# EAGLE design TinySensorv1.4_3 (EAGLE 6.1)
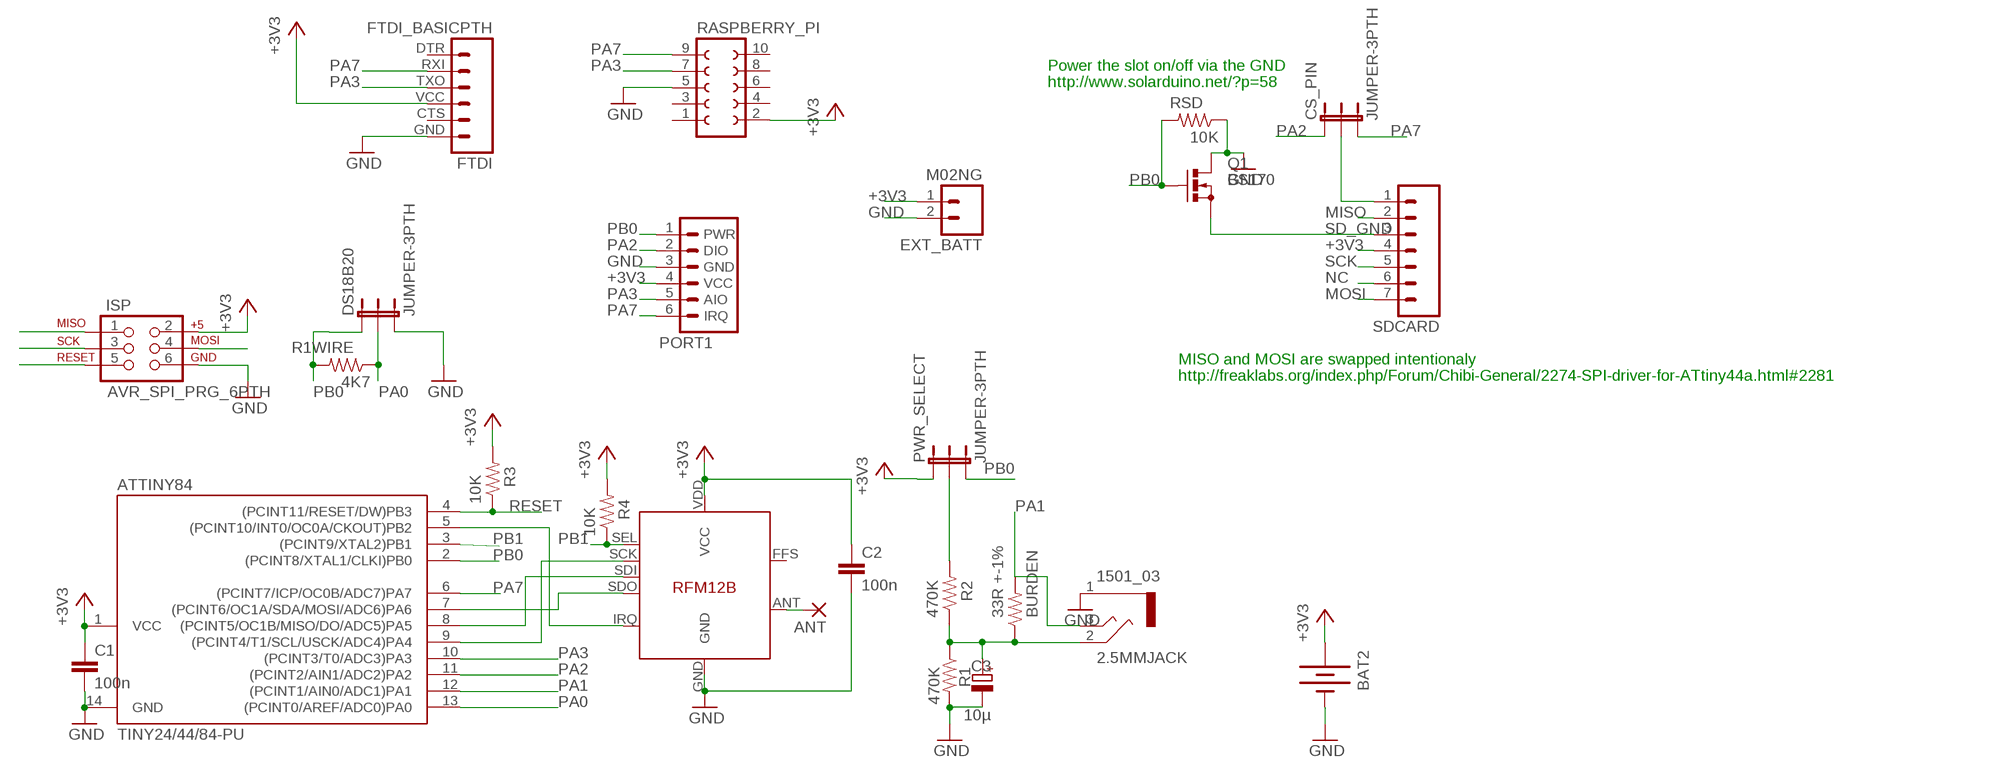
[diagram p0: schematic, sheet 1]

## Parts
2.5MMJACK  1501_03  [1501_03]
ANT  1,6/0,8  [1,6/0,8]
ATTINY84  TINY24/44/84-PU  [DIL14]
BAT2  BATTERY20PTH  [BATTCOM_20MM_PTH]
BURDEN  33R +-1%  RESISTORAXIAL-0.3  [AXIAL-0.3]
C1  100n  C-EU025-024X044  [C025-024X044]
C2  100n  C-EU025-024X044  [C025-024X044]
C3  10µ  CPOL-EUE2.5-6  [E2,5-6]
CS_PIN  JUMPER-3PTH  [1X03]
DS18B20  JUMPER-3PTH  [1X03]
EXT_BATT  M02NG  [1X02]
FTDI  FTDI_BASICPTH  [FTDI_BASIC]
ISP  AVR_SPI_PRG_6PTH  [2X3]
PORT1  JEEPORT-FEMALE  [1X06_FEMALE_LOCK.010]
PWR_SELECT  JUMPER-3PTH  [1X03]
Q1  BS170  [SOT54E]
R1  470K  RESISTORAXIAL-0.3  [AXIAL-0.3]
R1WIRE  4K7  RESISTORAXIAL-0.3  [AXIAL-0.3]
R2  470K  RESISTORAXIAL-0.3  [AXIAL-0.3]
R3  10K  RESISTORAXIAL-0.3  [AXIAL-0.3]
R4  10K  RESISTORAXIAL-0.3  [AXIAL-0.3]
RASPBERRY_PI  FE05-2  [FE05-2]
RFM12B  RFM12B  [RFM12B]
RSD  10K  RESISTORAXIAL-0.3  [AXIAL-0.3]
SDCARD  M07LOCK  [1X07_LOCK]

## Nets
+3V3 [power]: ATTINY84.1(VCC) BAT2.1(+) C1.1 C2.1 EXT_BATT.1 FTDI.VCC ISP.2 PORT1.4(VCC) PWR_SELECT.1 R3.P$2 R4.P$2 RASPBERRY_PI.2 RFM12B.VDD(VCC) SDCARD.4
GND [power]: 2.5MMJACK.1 ATTINY84.14(GND) BAT2.2(-) C1.2 C2.2 C3.- DS18B20.3 EXT_BATT.2 FTDI.GND ISP.6 PORT1.3(GND) Q1.D R1.P$2 RASPBERRY_PI.5 RFM12B.GND RSD.P$1
MISO: ATTINY84.8((PCINT5/OC1B/MISO/DO/ADC5)PA5) ISP.1 RFM12B.SDI SDCARD.2
MOSI: ATTINY84.7((PCINT6/OC1A/SDA/MOSI/ADC6)PA6) ISP.4 RFM12B.SDO SDCARD.7
N$1: PWR_SELECT.2 R2.P$2
N$3: CS_PIN.2 SDCARD.1
N$6 [power]: ANT.1(P) RFM12B.ANT
N$10: 2.5MMJACK.2 BURDEN.P$1 C3.+ R1.P$1 R2.P$1
NC: SDCARD.6
PA0: ATTINY84.13((PCINT0/AREF/ADC0)PA0) DS18B20.2 R1WIRE.P$1
PA1: 2.5MMJACK.3 ATTINY84.12((PCINT1/AIN0/ADC1)PA1) BURDEN.P$2
PA2: ATTINY84.11((PCINT2/AIN1/ADC2)PA2) CS_PIN.1 PORT1.2(DIO)
PA3: ATTINY84.10((PCINT3/T0/ADC3)PA3) FTDI.TXO PORT1.5(AIO) RASPBERRY_PI.7
PA7: ATTINY84.6((PCINT7/ICP/OC0B/ADC7)PA7) CS_PIN.3 FTDI.RXI PORT1.6(IRQ) RASPBERRY_PI.9
PB0: ATTINY84.2((PCINT8/XTAL1/CLKI)PB0) DS18B20.1 PORT1.1(PWR) PWR_SELECT.3 Q1.G R1WIRE.P$2 RSD.P$2
PB1: ATTINY84.3((PCINT9/XTAL2)PB1) R4.P$1 RFM12B.SEL
PB2: ATTINY84.5((PCINT10/INT0/OC0A/CKOUT)PB2) RFM12B.IRQ
RESET: ATTINY84.4((PCINT11/RESET/DW)PB3) ISP.5 R3.P$1
SCK: ATTINY84.9((PCINT4/T1/SCL/USCK/ADC4)PA4) ISP.3 RFM12B.SCK SDCARD.5
SD_GND: Q1.S SDCARD.3
Unconnected: FTDI.CTS FTDI.DTR RASPBERRY_PI.1 RASPBERRY_PI.3 RASPBERRY_PI.4 RASPBERRY_PI.6 RASPBERRY_PI.8 RASPBERRY_PI.10 RFM12B.FFS

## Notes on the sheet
- Power the slot on/off via the GND
- http://www.solarduino.net/?p=58
- MISO and MOSI are swapped intentionaly
- http://freaklabs.org/index.php/Forum/Chibi-General/2274-SPI-driver-for-ATtiny44a.html#2281

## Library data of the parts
2.5MMJACK = con-lumberg:1501_03: Klinkensteckverbinder nach JISC 6560, 2,5 mm Jack connectors according to JISC 6560, 2.5 mm Source: http://www.lumberg.com/Produkte/PDFs/1501_03.pdf; OC_FARNELL: 1200127; OC_NEWARK: unknown
ANT = JeeLabs:1,6/0,8: THROUGH-HOLE PAD
ATTINY84 = avr-7:TINY24/44/84
BAT2 = SparkFun:BATTERY: Battery Holders
BURDEN R1 R1WIRE R2-R4 RSD = SparkFun:RESISTOR: Resistor
C1 C2 = rcl:C-EU: CAPACITOR, European symbol
C3 = rcl:CPOL-EU: POLARIZED CAPACITOR, European symbol
CS_PIN DS18B20 PWR_SELECT = SparkFun:JUMPER-3
EXT_BATT = SparkFun:M02NG
FTDI = SparkFun:FTDI_BASIC: FTDI Basic: 3.3V and 5V
ISP = SparkFun:AVR_SPI_PRG_6: AVR ISP 6 Pin This is the reduced ISP connector for AVR programming. Common on Arduino. This footprint will take up less PCB space and can be used with a 10-pin to 6-pin adapter such as SKU: BOB-08508
PORT1 = JeeParts:JEEPORT: PIN HEADER
Q1 = transistor-small-signal:BS170: N-CHANNEL MOS FET
RASPBERRY_PI = con-lsta:FE05-2: FEMALE HEADER; OC_FARNELL: unknown; OC_NEWARK: unknown
RFM12B = JeeLabs:RFM12B
SDCARD = SparkFun:M07: Header 7 Standard 7-pin 0.1" header. Use with straight break away headers (SKU : PRT-00116), right angle break away headers (PRT-00553), swiss pins (PRT-00743), machine pins (PRT-00117), and female headers (PRT-00115). NOTES ON THE VARIANTS LOCK and LOCK_LONGPADS... This footprint was designed to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

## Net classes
0 default: width 0.356 mm, drill 0.356 mm, clearance 0.356 mm
1 power: width 0.406 mm, drill 0.356 mm, clearance 0.406 mm

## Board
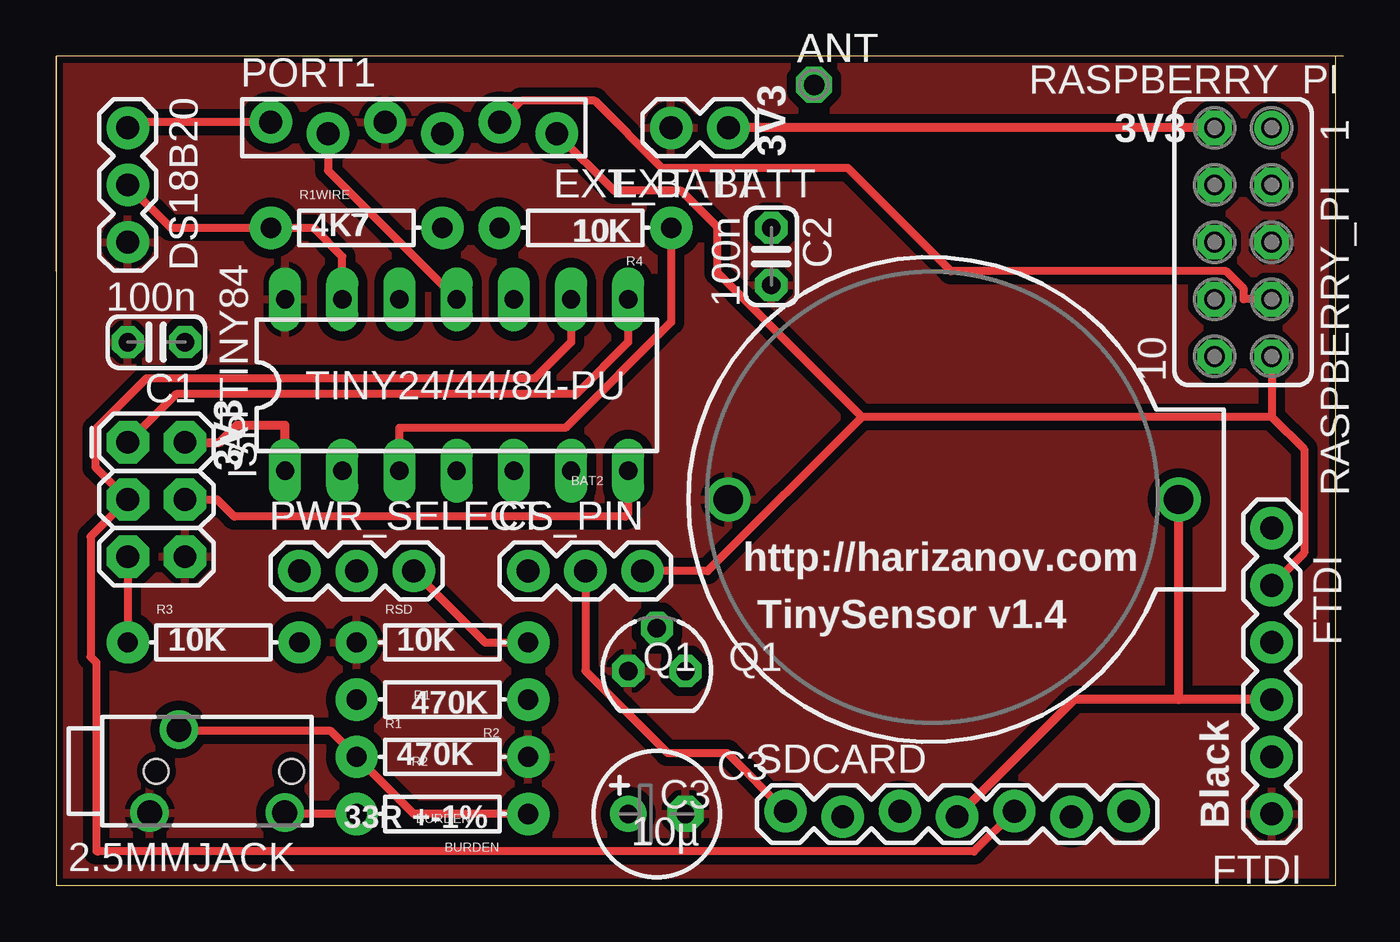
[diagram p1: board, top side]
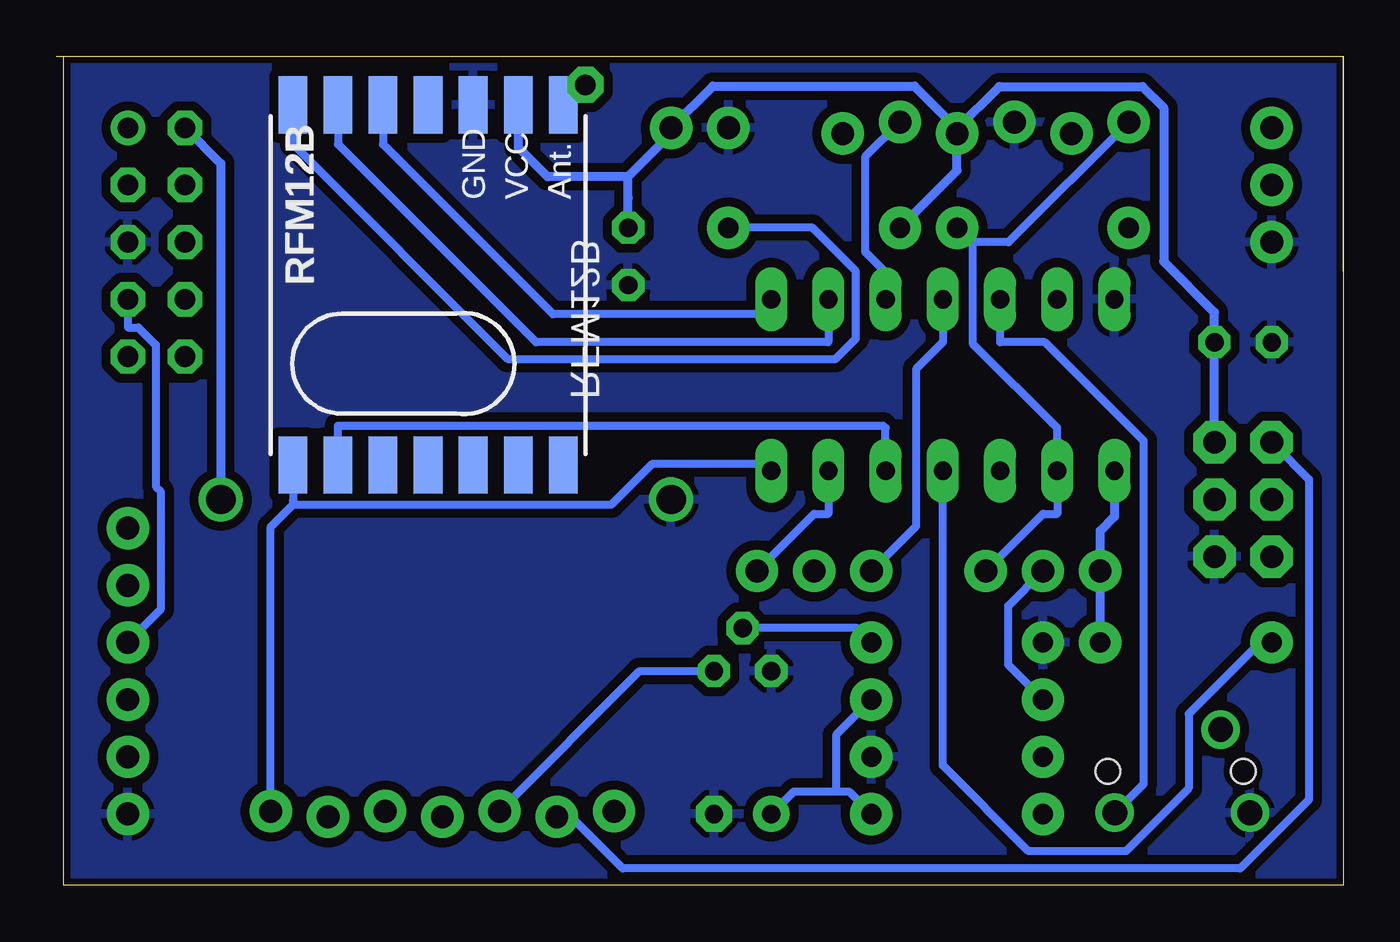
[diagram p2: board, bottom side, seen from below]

Size 57.15 x 36.83 mm. Coordinates in mm from the lower left corner, seen from the top.
Outline: 56.82,36.82 56.82,0 0,0 0,27.3
Outline: 0,27.3 0,36.83
Outline: 0,36.83 0,27.3
Outline: 57.15,36.83 0,36.83
Copper layers (1*16): Top 0.035mm / dielectric 1.5mm / Bottom 0.035mm
Design rules: minimum track width 12mil, minimum drill 24mil, track to track 12mil, track to pad 12mil, pad to pad 12mil, via to via 14mil, smd to smd 10mil, copper to edge 12mil, drill to drill 8mil, minimum pad ring 12mil, minimum via ring 8mil, stop-mask expansion 4mil, vias tented up to drill 0mil, thermal gap 10mil

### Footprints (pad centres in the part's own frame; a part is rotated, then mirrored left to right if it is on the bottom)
1501_03 = drill 1.1 pad 1.7: 1 -1.85,0.3; 2 1.85,-1; 3 -1.85,-5.7 | hole 1.1: 0,0; 0,-6
1,6/0,8 = drill 0.9 pad 1.6 octagon: 1 0,0
DIL14 = drill 0.813 long: 1 -7.62,-3.81; 2 -5.08,-3.81; 3 -2.54,-3.81; 4 0,-3.81; 5 2.54,-3.81; 6 5.08,-3.81; 7 7.62,-3.81; 8 7.62,3.81; 9 5.08,3.81; 10 2.54,3.81; 11 0,3.81; 12 -2.54,3.81; 13 -5.08,3.81; 14 -7.62,3.81
BATTCOM_20MM_PTH = drill 1.3: 1 20,0; 2 0,0
AXIAL-0.3 = drill 0.9 pad 1.88: P$1 -3.81,0; P$2 3.81,0
C025-024X044 = drill 0.813 octagon: 1 -1.27,0; 2 1.27,0
E2,5-6 = drill 0.813 pad 1.6: + -1.27,0 | drill 0.813 pad 1.6 octagon: - 1.27,0
1X03 = drill 1.016 pad 1.88: 1 0,0; 2 2.54,0; 3 5.08,0
1X02 = drill 1.016 pad 1.88: 1 0,0; 2 2.54,0
FTDI_BASIC = drill 1.016 pad 1.88: CTS 10.16,0; DTR 0,0; GND 12.7,0; RXI 2.54,0; TXO 5.08,0; VCC 7.62,0
2X3 = drill 1.016 pad 1.88 octagon: 1 0,0; 2 0,2.54; 3 2.54,0; 4 2.54,2.54; 5 5.08,0; 6 5.08,2.54
1X06_FEMALE_LOCK.010 = drill 1.016 pad 1.88: 1 0,0.254; 2 2.54,-0.254; 3 5.08,0.254; 4 7.62,-0.254; 5 10.16,0.254; 6 12.7,-0.254
SOT54E = drill 0.813 octagon: D -1.27,0; G 0,1.905; S 1.27,0
FE05-2 = drill 0.914: 1 -5.08,1.27 | drill 0.914 octagon: 2 -5.08,-1.27; 3 -2.54,1.27; 4 -2.54,-1.27; 5 0,1.27; 6 0,-1.27; 7 2.54,1.27; 8 2.54,-1.27; 9 5.08,1.27; 10 5.08,-1.27
RFM12B = smd 2.54 x 1.27: ANT 8,-6; FFS -8,2; GND 8,-2; IRQ -8,4; P$8 -8,0; P$9 -8,-2; P$10 -8,-4; P$12 -8,-6; P$16 8,0; SCK 8,4; SDI 8,2; SDO -8,6; SEL 8,6; VDD 8,-4
1X07_LOCK = drill 1.016 pad 1.88: 1 0,0.127; 2 2.54,-0.127; 3 5.08,0.127; 4 7.62,-0.127; 5 10.16,0.127; 6 12.7,-0.127; 7 15.24,0.127

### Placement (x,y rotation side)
2.5MMJACK  4.45,5.08 90 top
ANT  33.66,35.56 0 top
ATTINY84  17.78,22.23 0 top
BAT2  29.84,17.14 0 top
BURDEN  17.14,3.17 180 top
C1  4.45,24.13 180 top
C2  31.75,27.94 270 top
C3  26.67,3.17 0 top
CS_PIN  20.95,13.97 0 top
DS18B20  3.17,33.66 270 top
EXT_BATT  29.84,33.66 180 top
FTDI  53.98,15.88 270 top
ISP  3.17,19.68 270 top
PORT1  9.53,33.66 0 top
PWR_SELECT  10.79,13.97 0 top
Q1  26.67,9.53 0 top
R1  17.14,5.71 0 top
R1WIRE  13.34,29.21 0 top
R2  17.14,8.26 180 top
R3  6.99,10.79 0 top
R4  23.5,29.21 180 top
RASPBERRY_PI  52.7,28.57 270 top
RFM12B  40.64,26.67 90 bottom
RSD  17.14,10.79 0 top
SDCARD  32.38,3.17 0 top

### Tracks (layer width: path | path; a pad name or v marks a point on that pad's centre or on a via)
+3V3
  Top 0.406: RASPBERRY_PI.2 EXT_BATT.1 | 49.84,8.26 45.21,8.26 SDCARD.4 | FTDI.VCC 49.84,8.26 | 49.84,8.26 BAT2.1 | ISP.2 7.26,19.68 8.03,20.45 10.16,20.45 ATTINY84.1
  Bottom 0.406: 31.75,31.48 35.33,31.48 36.64,32.79 RFM12B.VDD | 31.75,31.48 29.84,33.39 EXT_BATT.1 28,35.5 19.03,35.5 17.14,33.62 | 31.75,31.48 31.75,30.53 C2.1 | 17.14,33.62 PORT1.4 17.14,31.75 R4.P$2 | 17.14,33.62 15.27,35.49 8.91,35.49 7.97,34.55 7.97,27.71 5.71,25.45 C1.1 ISP.2 | ATTINY84.1 10.16,16.38 10.79,15.75 PWR_SELECT.1 R3.P$2 | RASPBERRY_PI.2 49.84,32.06 BAT2.1
GND
  pour Bottom: -1.27,38.1 58.42,38.1 58.42,-1.27 -1.27,-1.27
  pour Top: -2.54,39.37 60.96,39.37 60.96,-2.54 -2.54,-2.54
MISO
  Top 0.356: ISP.1 5.32,21.83 23.1,21.83 25.4,24.13 ATTINY84.8
  Bottom 0.356: RFM12B.SDI 42.64,32.92 35.1,25.37 26.06,25.37 ATTINY84.8 | SDCARD.2 34.8,3.05 34.29,3.05 32,0.76 4.57,0.76 1.52,3.81 1.52,18.03 3.05,19.56 ISP.1
MOSI
  Top 0.356: ISP.4 7.14,17.14 7.9,16.38 25.27,16.38 25.4,16.51 ATTINY84.7
  Bottom 0.356: 46.64,16.92 32.5,16.92 30.67,18.74 25.73,18.74 ATTINY84.7 | 46.64,16.92 46.64,17.09 RFM12B.SDO | SDCARD.7 47.62,15.93 46.64,16.92
N$1
  Bottom 0.356: R2.P$2 14.88,9.8 14.88,12.43 PWR_SELECT.2
N$3
  Top 0.356: CS_PIN.2 23.5,9.54 27.14,5.89 29.8,5.89 SDCARD.1
N$6
  Bottom 0.406: RFM12B.ANT 34.55,34.67 ANT.1
N$10
  Top 0.356: BURDEN.P$1 15.88,3.17 R1.P$1 12.19,6.86 5.59,6.86 2.5MMJACK.2
  Bottom 0.356: 22.52,4.18 21.96,4.18 BURDEN.P$1 | C3.+ 24.4,4.18 22.52,4.18 | R2.P$1 22.52,6.69 22.52,4.18
PA0
  Top 0.356: ATTINY84.13 12.7,27.94 11.43,29.21 R1WIRE.P$1 5.08,29.21 DS18B20.2
PA1
  Top 0.356: BURDEN.P$2 10.2,3.17 2.5MMJACK.3
  Bottom 0.356: ATTINY84.12 15.24,24.13 13.25,24.13 8.86,19.74 8.86,4.51 2.5MMJACK.3
PA2
  Top 0.356: PORT1.2 12.06,31.75 ATTINY84.11
  Bottom 0.356: ATTINY84.11 17.78,24.13 18.97,22.94 18.97,15.95 CS_PIN.1
PA3
  Top 0.356: PORT1.5 20.63,34.86 23.92,34.86 26.91,31.86 35.15,31.86 39.74,27.28 51.95,27.28 52.73,26.5 52.73,26.04 RASPBERRY_PI.7
  Bottom 0.356: RASPBERRY_PI.7 53.98,24.79 53.51,24.79 52.73,24.01 52.73,17.73 52.52,17.51 52.52,12.25 FTDI.TXO | PORT1.5 21.23,32.36 21.23,28.15 20.32,27.24 ATTINY84.10
PA7
  Top 0.356: 53.98,20.82 55.41,19.38 55.41,14.77 FTDI.RXI | 53.98,20.82 53.98,22.25 53.98,22.87 RASPBERRY_PI.9 | 53.98,20.82 35.77,20.82 | 35.77,20.82 | 35.77,20.82 29.36,27.23 29.36,29.24 27.74,30.85 24.77,30.85 PORT1.6 | 35.77,20.82 28.93,13.97 CS_PIN.3
  Bottom 0.356: ATTINY84.6 22.86,16.51 23.5,16.51 CS_PIN.3
PB0
  Top 0.356: PWR_SELECT.3 19.05,10.79 RSD.P$2 | PORT1.1 3.43,33.91 DS18B20.1
  Bottom 0.356: RSD.P$2 21.59,11.43 Q1.G | 16.46,28.57 16.51,28.57 R1WIRE.P$2 | PORT1.1 14.86,28.57 16.46,28.57 | 16.46,28.57 16.46,24.08 12.7,20.32 ATTINY84.2 12.7,16.51 13.34,16.51 PWR_SELECT.3
PB1
  Top 0.356: ATTINY84.3 15.24,20.32 22.61,20.32 27.3,25.02 R4.P$1
  Bottom 0.356: RFM12B.SEL 46.64,32.92 37.11,23.39 22.54,23.39 21.64,24.29 21.64,27.29 23.56,29.21 R4.P$1
PB2
  Bottom 0.356: ATTINY84.5 20.32,20.32 20.42,20.42 44.64,20.42 RFM12B.IRQ
RESET
  Top 0.356: ISP.5 R3.P$1
  Bottom 0.356: ATTINY84.4 17.78,18.29 17.78,5.33 13.97,1.52 9.65,1.52 6.86,4.32 6.86,7.62 3.81,10.67 3.3,10.67 R3.P$1
SCK
  Top 0.356: ATTINY84.9 22.86,24.13 21.27,22.54 4.01,22.54 1.75,20.27 1.75,18.57 ISP.3 1.78,15.75 | SDCARD.5 40.76,1.52 1.84,1.52 1.78,1.52 1.78,9.91 1.52,10.16 1.52,15.49 1.78,15.75 | 1.75,15.72 1.78,15.75
  Bottom 0.356: RFM12B.SCK 44.64,32.92 35.85,24.13 22.86,24.13 ATTINY84.9
SD_GND
  Bottom 0.356: SDCARD.3 31.24,9.53 Q1.S

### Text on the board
_tsilk: ANT | DS18B20 | PORT1 | RASPBERRY_PI | 3V3 | 3V3 | EXT_BATT | 10K | 100n | C2 | 4K7 | 100n | C1 | TINY24/44/84-PU | 3V3 | PWR_SELECT | CS_PIN | 3V3 | http://harizanov.com | TinySensor v1.4 | 10K | 10K | Q1 | R1 | R2 | SDCARD | BURDEN | C3 | Black | 10µ | FTDI
_bsilk: Ant. | VCC | GND | RFM12B | RFM12B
